|   IBIS model for TI AM261
[IBIS Ver]   5.1
[Disclaimer]   Please be aware that in the absence of a written agreement
|   Texas Instruments(TI) assumes no liability for:
|   (1) The accuracy of the IBIS models provided to your company,
|   however, the IBIS model is compliant to industry standard
|   IQ Level 2a.  Refer to IBIS Quality Section below for
|   for full details.
|   (2) The proper functioning of these Models in your design
|   or for any resulting applications
|   (3) Infringement of patents, copyrights or intellectual
|   property rights resulting from your use of these
|   models.
|   TI provides IBIS Models as a service to our customers and
|   therefore reserves the right to limit distribution of the
|   Models.  The information is subject to change without notice.
[File Name]  znc.ibs
[File Rev]   0.1
|   -Initial version
|   -Updated Package model
[Date]   10 October 2024
[Source]   Texas Instruments Incorporated
[Copyright]   Property of Texas Instruments Incorporated.
|   Unauthorized reproduction and/or distribution is strictly.
|   prohibited.
|   This product is protected under copyright law and trade
|   secret law as an unpublished work.
|   Created 2012,(C) Copyright 1999-2012,
|   Texas Instruments Incorporated., All Rights Reserved.
|   These commodities are under the U.S. Government
|   distribution license control. As such,they are not to be
|   re-exported without the prior approval of the U.S.
|   Department of Commerce.
[Notes]
   ADC pins are marked as NC
   USB pins are marked as NC
   Clock pins are marked as NC
   nReset pin marked as NC
|   Revision History
|   GERNERAL COMMENT: All IBIS Quality Notes below reflect latest release
|   and version of IBIS File
|   File passes ibischk6.0 with 0 errors and 35 warnings
|   Component AM261
[Component] AM261
[Manufacturer] TEXAS INSTRUMENTS
[Package Model] AM261_ZNC
[Package]
|   typ   min   max
R_pkg   0.1315   0.055671   0.23353
L_pkg   2.085e-9   9.776e-10   4.208e-9
C_pkg   2.503e-13   1.668e-13   9.865e-13
[Pin]   Signal_name   model_name
E6   VDD   POWER
E8   VDD   POWER
E10   VDD   POWER
E12   VDD   POWER
E14   VDD   POWER
F5   VDD   POWER
F15   VDD   POWER
H5   VDD   POWER
H15   VDD   POWER
K5   VDD   POWER
K15   VDD   POWER
M5   VDD   POWER
M15   VDD   POWER
P5   VDD   POWER
P15   VDD   POWER
R6   VDD   POWER
R15   VDD   POWER
T6   VDD   POWER
U9   VDDA18_LDO   POWER
U7   VDDA18_OSC_PLL   POWER
U3   VDDA18_USB   POWER
T10   VDDA33   POWER
T12   VDDA33   POWER
R3   VDDA33_USB   POWER
C11   VDDAR2   POWER
G3   VDDAR3   POWER
D6   VDDS18   POWER
D10   VDDS18   POWER
D14   VDDS18   POWER
H4   VDDS18   POWER
H16   VDDS18   POWER
L3   VDDS18   POWER
M16   VDDS18   POWER
T16   VDDS18   POWER
V4   VDDS18_LDO   POWER
C15   VDDSHV_A   POWER
D8   VDDSHV_A   POWER
D12   VDDSHV_A   POWER
F4   VDDSHV_A   POWER
F16   VDDSHV_A   POWER
K16   VDDSHV_A   POWER
P4   VDDSHV_B   POWER
T14   VDDSHV_C   POWER
K4   VDDSHV_D   POWER
M4   VDDSHV_D   POWER
P16   VDDSHV_E   POWER
U5   VDDSHV_F   POWER
T8   VDD_TEMP   NC
J17   VNWA   POWER
N3   VPP   POWER
W12   ADC0_AIN0   NC
V12   ADC0_AIN1   NC
V13   ADC0_AIN2   NC
U11   ADC0_AIN3   NC
W13   ADC0_AIN4   NC
U13   ADC0_AIN5   NC
W14   ADC0_AIN6   NC
W8   ADC2_AIN0   NC
V9   ADC2_AIN1   NC
V6   ADC2_AIN2   NC
V7   ADC2_AIN3   NC
W9   ADC2_AIN4   NC
V8   ADC2_AIN5   NC
W7   ADC2_AIN6   NC
U15   ADC_CAL0   NC
V11   ADC_VREFHI_G0   NC
V10   ADC_VREFHI_G1   NC
W11   ADC_VREFLO_G0   NC
W10   ADC_VREFLO_G1   NC
W5   ATESTV1   NC
W6   DAC_OUT   NC
V14   DAC_VREF0   NC
R1   GPIO0   bc1833dv40dcpbfbp18ll_rxll_ssdlv
R2   GPIO1   bc1833dv40dcpbfbp18ll_rxll_ssdlv
M2   GPIO2   bc1833dv40dcpbfbp18ll_rxll_ssdlv
N2   GPIO3   bc1833dv40dcpbfbp18ll_ssdlv
N1   GPIO4   bc1833dv40dcpbfbp18ll_ssdlv
P2   GPIO5   bc1833dv40dcpbfbp18ll_rxll_ssdlv
P1   GPIO6   bc1833dv40dcpbfbp18ll_rxll_ssdlv
K2   GPIO7   bc1833dv40dcpbfbp18ll_rxll_ssdlv
L1   GPIO8   bc1833dv40dcpbfbp18ll_rxll_ssdlv
J2   GPIO9   bc1833dv40dcpbfbp18ll_rxll_ssdlv
K1   GPIO10   bc1833dv40dcpbfbp18ll_rxll_ssdlv
C13   GPIO11   bc1833dv40dcpbfbp18ll_rxll_ssdlh
A12   GPIO12   bc1833dv40dcpbfbp18ll_ssdlh
B12   GPIO13   bc1833dv40dcpbfbp18ll_ssdlh
B11   GPIO14   bc1833dv40dcpbfbp18ll_rxll_ssdlh
A11   GPIO19   bc1833dv40dcpbfbp18ll_rxll_ssdlh
B10   GPIO20   bc1833dv40dcpbfbp18ll_rxll_ssdlh
A10   GPIO21   bc1833dv40dcpbfbp18ll_rxll_ssdlh
B9   GPIO22   bc1833dv40dcpbfbp18ll_rxll_ssdlh
C9   GPIO25   bc1833dv40dcpbfbp18ll_rxll_ssdlh
A9   GPIO26   bc1833dv40dcpbfbp18ll_rxll_ssdlh
A8   GPIO27   bc1833dv40dcpbfbp18ll_rxll_ssdlh
B8   GPIO28   bc1833dv40dcpbfbp18ll_rxll_ssdlh
V19   GPIO29   bc1833dv40dcpbfbp18ll_rxll_ssdlv_135u
U17   GPIO30   bc1833dv40dcpbfbp18ll_rxll_ssdlv_135u
W17   GPIO31   bc1833dv40dcpbfbp18ll_rxll_ssdlh
V17   GPIO32   bc1833dv40dcpbfbp18ll_rxll_ssdlh
W18   GPIO33   bc1833dv40dcpbfbp18ll_rxll_ssdlh
V18   GPIO34   bc1833dv40dcpbfbp18ll_rxll_ssdlv_135u
R18   GPIO35   bc1833dv40dcpbfbp18ll_rxll_ssdlv_135u
T19   GPIO36   bc1833dv40dcpbfbp18ll_rxll_ssdlv_135u
U18   GPIO37   bc1833dv40dcpbfbp18ll_rxll_ssdlv_135u
U19   GPIO38   bc1833dv40dcpbfbp18ll_rxll_ssdlv_135u
R17   GPIO39   bc1833dv40dcpbfbp18ll_rxll_ssdlv_135u
T18   GPIO40   bc1833dv40dcpbfbp18ll_rxll_ssdlv_135u
P18   GPIO41   bc1833dv40dcpbfbp18ll_rxll_ssdlv_135u
R19   GPIO42   bc1833dv40dcpbfbp18ll_rxll_ssdlv_135u
B5   GPIO43   bc1833dv40dcpbfbp18ll_rxll_ssdlh_135u
A6   GPIO44   bc1833dv40dcpbfbp18ll_rxll_ssdlh_135u
A5   GPIO45   bc1833dv40dcpbfbp18ll_rxll_ssdlh_135u
A4   GPIO46   bc1833dv40dcpbfbp18ll_rxll_ssdlh_135u
A3   GPIO47   bc1833dv40dcpbfbp18ll_rxll_ssdlh_135u
B4   GPIO48   bc1833dv40dcpbfbp18ll_rxll_ssdlh_135u
A2   GPIO49   bc1833dv40dcpbfbp18ll_rxll_ssdlh_135u
B2   GPIO50   bc1833dv40dcpbfbp18ll_rxll_ssdlv
B1   GPIO51   bc1833dv40dcpbfbp18ll_rxll_ssdlv
B3   GPIO52   bc1833dv40dcpbfbp18ll_rxll_ssdlv
C2   GPIO53   bc1833dv40dcpbfbp18ll_rxll_ssdlv
C1   GPIO54   bc1833dv40dcpbfbp18ll_rxll_ssdlv
E3   GPIO55   bc1833dv40dcpbfbp18ll_rxll_ssdlv
E2   GPIO56   bc1833dv40dcpbfbp18ll_rxll_ssdlv
D2   GPIO57   bc1833dv40dcpbfbp18ll_rxll_ssdlv
D1   GPIO58   bc1833dv40dcpbfbp18ll_rxll_ssdlv
E1   GPIO59   bc1833dv40dcpbfbp18ll_rxll_ssdlv
F1   GPIO60   bc1833dv40dcpbfbp18ll_rxll_ssdlv
F2   GPIO61   bc1833dv40dcpbfbp18ll_rxll_ssdlv
G1   GPIO62   bc1833dv40dcpbfbp18ll_rxll_ssdlv
G2   GPIO67   bc1833dv40dcpbfbp18ll_rxll_ssdlv
H1   GPIO68   bc1833dv40dcpbfbp18ll_rxll_ssdlv
H2   GPIO69   bc1833dv40dcpbfbp18ll_rxll_ssdlv
J1   GPIO70   bc1833dv40dcpbfbp18ll_rxll_ssdlv
V15   GPIO71   bc1833dv40dcpbfbp18ll_rxll_ssdlh
W15   GPIO72   bc1833dv40dcpbfbp18ll_rxll_ssdlh
W16   GPIO73   bc1833dv40dcpbfbp18ll_rxll_ssdlh
V16   GPIO74   bc1833dv40dcpbfbp18ll_rxll_ssdlh
L2   GPIO75   bc1833dv40dcpbfbp18ll_rxll_ssdlv
M1   GPIO76   bc1833dv40dcpbfbp18ll_rxll_ssdlv
N17   GPIO85   bc1833dv40dcpbfbp18ll_rxll_ssdlv_135u
P19   GPIO86   bc1833dv40dcpbfbp18ll_rxll_ssdlv_135u
G17   GPIO87   bc1833dv40dcpbfbp18ll_rxll_ssdlv_135u
J18   GPIO89   bc1833dv40dcpbfbp18ll_rxll_ssdlv_135u
G19   GPIO90   bc1833dv40dcpbfbp18ll_rxll_ssdlv_135u
L18   GPIO91   bc1833dv40dcpbfbp18ll_rxll_ssdlv_135u
J19   GPIO92   bc1833dv40dcpbfbp18ll_rxll_ssdlv_135u
M18   GPIO93   bc1833dv40dcpbfbp18ll_rxll_ssdlv_135u
L19   GPIO94   bc1833dv40dcpbfbp18ll_rxll_ssdlv_135u
K19   GPIO95   bc1833dv40dcpbfbp18ll_rxll_ssdlv_135u
L17   GPIO96   bc1833dv40dcpbfbp18ll_rxll_ssdlv_135u
K18   GPIO97   bc1833dv40dcpbfbp18ll_rxll_ssdlv_135u
M19   GPIO98   bc1833dv40dcpbfbp18ll_rxll_ssdlv_135u
N18   GPIO99   bc1833dv40dcpbfbp18ll_rxll_ssdlv_135u
N19   GPIO100   bc1833dv40dcpbfbp18ll_rxll_ssdlv_135u
H19   GPIO101   bc1833dv40dcpbfbp18ll_rxll_ssdlv_135u
H18   GPIO102   bc1833dv40dcpbfbp18ll_rxll_ssdlv_135u
E18   GPIO103   bc1833dv40dcpbfbp18ll_rxll_ssdlv_135u
C19   GPIO106   bc1833dv40dcpbfbp18ll_rxll_ssdlv_135u
D19   GPIO107   bc1833dv40dcpbfbp18ll_rxll_ssdlv_135u
E19   GPIO108   bc1833dv40dcpbfbp18ll_rxll_ssdlv_135u
G18   GPIO109   bc1833dv40dcpbfbp18ll_rxll_ssdlv_135u
F18   GPIO110   bc1833dv40dcpbfbp18ll_rxll_ssdlv_135u
E17   GPIO111   bc1833dv40dcpbfbp18ll_rxll_ssdlv_135u
F19   GPIO112   bc1833dv40dcpbfbp18ll_rxll_ssdlv_135u
B18   GPIO113   bc1833dv40dcpbfbp18ll_rxll_ssdlv_135u
A18   GPIO114   bc1833dv40dcpbfbp18ll_rxll_ssdlv_135u
D18   GPIO115   bc1833dv40dcpbfbp18ll_rxll_ssdlv_135u
C18   GPIO116   bc1833dv40dcpbfbp18ll_rxll_ssdlv_135u
B19   GPIO117   bc1833dv40dcpbfbp18ll_rxll_ssdlv_135u
C17   GPIO118   bc1833dv40dcpbfbp18ll_rxll_ssdlv_135u
B16   GPIO119   bc1833dv40dcpbfbp18ll_rxll_ssdlh
B17   GPIO120   bc1833dv40dcpbfbp18ll_rxll_ssdlv_135u
T1   GPIO121   bc1833dv40dcpbfbp18ll_rxll_ssdlh
A17   GPIO126   bc1833dv40dcpbfbp18ll_rxll_ssdlh
A16   GPIO127   bc1833dv40dcpbfbp18ll_rxll_ssdlh
B15   GPIO130   bc1833dv40dcpbfbp18ll_rxll_ssdlh
A15   GPIO131   bc1833dv40dcpbfbp18ll_rxll_ssdlh
A14   GPIO132   bc1833dv40dcpbfbp18ll_rxll_ssdlh
B14   GPIO133   bc1833dv40dcpbfbp18ll_rxll_ssdlh
B13   GPIO134   bi2c1833dvfzp18_ssdlh
A13   GPIO135   bi2c1833dvfzp18_ssdlh
J3   GPIO138   bc1833dv40dcpbfbp18ll_rxll_ssdlv
V1   GPIO139   NC
U1   GPIO140   NC
T2   PORZ   ihhv1833dvhyp18ll_ssdhv
C5   SAFETY_ERRORN   bc1833dv40dcpbfbp18ll_ssdlh_135u
B6   TCK   iq1833dvtckpbfbp18ll_ssdhh_135u
C7   TDI   bc1833dv40dcpbfbp18ll_ssdlh_135u
A7   TDO   bc1833dv40dcpbfbp18ll_ssdlh_135u
W4   TEMPCAL   NC
B7   TMS   bc1833dv40dcpbfbp18ll_ssdlh_135u
V5   VSYS_MON   NC
C3   WARMRSTN   bc1833dv40dcpbfbp18ll_od_fs_cmphdl_ssdlv
W3   XTAL_XI   NC
W2   XTAL_XO   NC
A1   VSS   GND
A19   VSS   GND
D4   VSS   GND
D16   VSS   GND
E5   VSS   GND
E15   VSS   GND
F6   VSS   GND
F7   VSS   GND
F8   VSS   GND
F9   VSS   GND
F10   VSS   GND
F11   VSS   GND
F12   VSS   GND
F13   VSS   GND
F14   VSS   GND
G6   VSS   GND
G7   VSS   GND
G8   VSS   GND
G9   VSS   GND
G10   VSS   GND
G11   VSS   GND
G12   VSS   GND
G13   VSS   GND
G14   VSS   GND
H6   VSS   GND
H7   VSS   GND
H8   VSS   GND
H9   VSS   GND
H10   VSS   GND
H11   VSS   GND
H12   VSS   GND
H13   VSS   GND
H14   VSS   GND
J6   VSS   GND
J7   VSS   GND
J8   VSS   GND
J9   VSS   GND
J10   VSS   GND
J11   VSS   GND
J12   VSS   GND
J13   VSS   GND
J14   VSS   GND
K6   VSS   GND
K7   VSS   GND
K8   VSS   GND
K9   VSS   GND
K10   VSS   GND
K11   VSS   GND
K12   VSS   GND
K13   VSS   GND
K14   VSS   GND
L6   VSS   GND
L7   VSS   GND
L8   VSS   GND
L9   VSS   GND
L10   VSS   GND
L11   VSS   GND
L12   VSS   GND
L13   VSS   GND
L14   VSS   GND
M6   VSS   GND
M7   VSS   GND
M8   VSS   GND
M9   VSS   GND
M10   VSS   GND
M11   VSS   GND
M12   VSS   GND
M13   VSS   GND
M14   VSS   GND
N6   VSS   GND
N7   VSS   GND
N8   VSS   GND
N9   VSS   GND
N10   VSS   GND
N11   VSS   GND
N12   VSS   GND
N13   VSS   GND
N14   VSS   GND
P6   VSS   GND
P7   VSS   GND
P8   VSS   GND
P9   VSS   GND
P10   VSS   GND
P11   VSS   GND
P12   VSS   GND
P13   VSS   GND
P14   VSS   GND
R5   VSS   GND
R8   VSS   GND
R14   VSS   GND
T4   VSS   GND
U2   VSS   GND
V2   VSS   GND
V3   VSS   GND
W1   VSS   GND
W19   VSS   GND
R10   VSSA   GND
R12   VSSA   GND
|   BC1833DV40DCPBFBP18LL_SSDLH
[Model Selector] bc1833dv40dcpbfbp18ll_ssdlh
|SC1 IS A SLEW RATE CONTROL PIN
|5% SUPPLY VARIATION MODES WITH 1.8V NOM SUPPLY
BC40D_H_PUPDOFF_5P_SC1_1P8  Cell operated at 1.8(nom)
|BC40D_H_PUPDOFF_5P_SC1_1P8; BUFFER WITH WEAK PULUP/PULLDOWN OFF AT 5% SUPPLY
|VARIATION WITH SC1=1 MEANING SLOW MODE OF OPERATION
BC40D_H_PD_ON_5P_!SC1_1P8  Cell operated at 1.8(nom)
|BC40D_H_PD_ON_5P_!SC1_1P8; BUFFER WITH WEAK_PULLDOWN_ON AT 5% SUPPLY
|VARIATION WITH SC1=0 MEANING FAST MODE OF OPERATION
BC40D_H_PD_ON_5P_SC1_1P8  Cell operated at 1.8(nom)
|BC40D_H_PD_ON_5P_SC1_1P8; BUFFER WITH WEAK_PULLDOWN_ON AT 5% SUPPLY
|VARIATION WITH SC1=1 MEANING SLOW MODE OF OPERATION
BC40D_H_PU_ON_5P_!SC1_1P8  Cell operated at 1.8(nom)
|BC40D_H_PU_ON_5P_!SC1_1P8; BUFFER WITH WEAK_PULLUP_ON AT 5% SUPPLY
|VARIATION WITH SC1=0 MEANING FAST MODE OF OPERATION
BC40D_H_PUPDOFF_5P_!SC1_1P8  Cell operated at 1.8(nom)
|BC40D_H_PUPDOFF_5P_!SC1_1P8; BUFFER WITH WEAK PULUP/PULLDOWN OFF AT 5% SUPPLY
|VARIATION WITH SC1=0 MEANING FAST MODE OF OPERATION
BC40D_H_PU_ON_5P_SC1_1P8  Cell operated at 1.8(nom)
|BC40D_H_PU_ON_5P_SC1_1P8; BUFFER WITH WEAK_PULLUP_ON AT 5% SUPPLY
|VARIATION WITH SC1=1 MEANING SLOW MODE OF OPERATION
|5% SUPPLY VARIATION MODES WITH 3.3V NOM SUPPLY
BC40D_H_PUPDOFF_5P_SC1_3P3  Cell operated at 3.3(nom)
|BC40D_H_PUPDOFF_5P_SC1_3P3; BUFFER WITH WEAK PULUP/PULLDOWN OFF AT 5% SUPPLY
|VARIATION WITH SC1=1 MEANING SLOW MODE OF OPERATION
BC40D_H_PD_ON_5P_!SC1_3P3  Cell operated at 3.3(nom)
|BC40D_H_PD_ON_5P_!SC1_3P3; BUFFER WITH WEAK_PULLDOWN_ON AT 5% SUPPLY
|VARIATION WITH SC1=0 MEANING FAST MODE OF OPERATION
BC40D_H_PD_ON_5P_SC1_3P3  Cell operated at 3.3(nom)
|BC40D_H_PD_ON_5P_SC1_3P3; BUFFER WITH WEAK_PULLDOWN_ON AT 5% SUPPLY
|VARIATION WITH SC1=1 MEANING SLOW MODE OF OPERATION
BC40D_H_PU_ON_5P_!SC1_3P3  Cell operated at 3.3(nom)
|BC40D_H_PU_ON_5P_!SC1_3P3; BUFFER WITH WEAK_PULLUP_ON AT 5% SUPPLY
|VARIATION WITH SC1=0 MEANING FAST MODE OF OPERATION
BC40D_H_PUPDOFF_5P_!SC1_3P3  Cell operated at 3.3(nom)
|BC40D_H_PUPDOFF_5P_!SC1_3P3; BUFFER WITH WEAK PULUP/PULLDOWN OFF AT 5% SUPPLY
|VARIATION WITH SC1=0 MEANING FAST MODE OF OPERATION
BC40D_H_PU_ON_5P_SC1_3P3  Cell operated at 3.3(nom)
|BC40D_H_PU_ON_5P_SC1_3P3; BUFFER WITH WEAK_PULLUP_ON AT 5% SUPPLY
|VARIATION WITH SC1=1 MEANING SLOW MODE OF OPERATION
| 10% SUPPLY VARIATION MODES WITH 1.8V NOM SUPPLY
BC40D_H_PUPDOFF_10P_SC1_1P8  Cell operated at 1.8(nom)
|BC40D_H_PUPDOFF_10P_SC1_1P8; BUFFER WITH WEAK PULUP/PULLDOWN OFF AT 10% SUPPLY
|VARIATION WITH SC1=1 MEANING SLOW MODE OF OPERATION
BC40D_H_PD_ON_10P_!SC1_1P8  Cell operated at 1.8(nom)
|BC40D_H_PD_ON_10P_!SC1_1P8; BUFFER WITH WEAK_PULLDOWN_ON AT 10% SUPPLY
|VARIATION WITH SC1=0 MEANING FAST MODE OF OPERATION
BC40D_H_PD_ON_10P_SC1_1P8  Cell operated at 1.8(nom)
|BC40D_H_PD_ON_10P_SC1_1P8; BUFFER WITH WEAK_PULLDOWN_ON AT 10% SUPPLY
|VARIATION WITH SC1=1 MEANING SLOW MODE OF OPERATION
BC40D_H_PU_ON_10P_!SC1_1P8  Cell operated at 1.8(nom)
|BC40D_H_PU_ON_10P_!SC1_1P8; BUFFER WITH WEAK_PULLUP_ON AT 10% SUPPLY
|VARIATION WITH SC1=0 MEANING FAST MODE OF OPERATION
BC40D_H_PUPDOFF_10P_!SC1_1P8  Cell operated at 1.8(nom)
|BC40D_H_PUPDOFF_10P_!SC1_1P8; BUFFER WITH WEAK PULUP/PULLDOWN OFF AT 10% SUPPLY
|VARIATION WITH SC1=0 MEANING FAST MODE OF OPERATION
BC40D_H_PU_ON_10P_SC1_1P8  Cell operated at 1.8(nom)
|BC40D_H_PU_ON_10P_SC1_1P8; BUFFER WITH WEAK_PULLUP_ON AT 10% SUPPLY
|VARIATION WITH SC1=1 MEANING SLOW MODE OF OPERATION
| 10% SUPPLY VARIATION MODES WITH 3.3V NOM SUPPLY
BC40D_H_PUPDOFF_10P_SC1_3P3  Cell operated at 3.3(nom)
|BC40D_H_PUPDOFF_10P_SC1_3P3; BUFFER WITH WEAK PULUP/PULLDOWN OFF AT 10% SUPPLY
|VARIATION WITH SC1=1 MEANING SLOW MODE OF OPERATION
BC40D_H_PD_ON_10P_!SC1_3P3  Cell operated at 3.3(nom)
|BC40D_H_PD_ON_10P_!SC1_3P3; BUFFER WITH WEAK_PULLDOWN_ON 10% SUPPLY
|VARIATION WITH SC1=0 MEANING FAST MODE OF OPERATION
BC40D_H_PD_ON_10P_SC1_3P3  Cell operated at 3.3(nom)
|BC40D_H_PD_ON_10P_SC1_3P3; BUFFER WITH WEAK_PULLDOWN_ON AT 10% SUPPLY
|VARIATION WITH SC1=1 MEANING SLOW MODE OF OPERATION
BC40D_H_PU_ON_10P_!SC1_3P3  Cell operated at 3.3(nom)
|BC40D_H_PU_ON_10P_!SC1_3P3; BUFFER WITH WEAK_PULLUP_ON AT 10% SUPPLY
|VARIATION WITH SC1=0 MEANING FAST MODE OF OPERATION
BC40D_H_PUPDOFF_10P_!SC1_3P3  Cell operated at 3.3(nom)
|BC40D_H_PUPDOFF_10P_!SC1_3P3; BUFFER WITH WEAK PULUP/PULLDOWN OFF AT 10% SUPPLY
|VARIATION WITH SC1=0 MEANING FAST MODE OF OPERATION
BC40D_H_PU_ON_10P_SC1_3P3  Cell operated at 3.3(nom)
|BC40D_H_PU_ON_10P_SC1_3P3; BUFFER WITH WEAK_PULLUP_ON AT 10% SUPPLY
|VARIATION WITH SC1=1 MEANING SLOW MODE OF OPERATION
|   BC1833DV40DCPBFBP18LL_SSDLV
[Model Selector] bc1833dv40dcpbfbp18ll_ssdlv
|SC1 IS A SLEW RATE CONTROL PIN
|5% SUPPLY VARIATION MODES WITH 1.8V NOM SUPPLY
BC40D_V_PUPDOFF_5P_SC1_1P8  Cell operated at 1.8(nom)
|BC40D_V_PUPDOFF_5P_SC1_1P8; BUFFER WITH WEAK PULUP/PULLDOWN OFF AT 5% SUPPLY
|VARIATION WITH SC1=1 MEANING SLOW MODE OF OPERATION
BC40D_V_PD_ON_5P_!SC1_1P8  Cell operated at 1.8(nom)
|BC40D_V_PD_ON_5P_!SC1_1P8; BUFFER WITH WEAK_PULLDOWN_ON AT 5% SUPPLY
|VARIATION WITH SC1=0 MEANING FAST MODE OF OPERATION
BC40D_V_PD_ON_5P_SC1_1P8  Cell operated at 1.8(nom)
|BC40D_V_PD_ON_5P_SC1_1P8; BUFFER WITH WEAK_PULLDOWN_ON AT 5% SUPPLY
|VARIATION WITH SC1=1 MEANING SLOW MODE OF OPERATION
BC40D_V_PU_ON_5P_!SC1_1P8  Cell operated at 1.8(nom)
|BC40D_V_PU_ON_5P_!SC1_1P8; BUFFER WITH WEAK_PULLUP_ON AT 5% SUPPLY
|VARIATION WITH SC1=0 MEANING FAST MODE OF OPERATION
BC40D_V_PUPDOFF_5P_!SC1_1P8  Cell operated at 1.8(nom)
|BC40D_V_PUPDOFF_5P_!SC1_1P8; BUFFER WITH WEAK PULUP/PULLDOWN OFF AT 5% SUPPLY
|VARIATION WITH SC1=0 MEANING FAST MODE OF OPERATION
BC40D_V_PU_ON_5P_SC1_1P8  Cell operated at 1.8(nom)
|BC40D_V_PU_ON_5P_SC1_1P8; BUFFER WITH WEAK_PULLUP_ON AT 5% SUPPLY
|VARIATION WITH SC1=1 MEANING SLOW MODE OF OPERATION
|5% SUPPLY VARIATION MODES WITH 3.3V NOM SUPPLY
BC40D_V_PUPDOFF_5P_SC1_3P3  Cell operated at 3.3(nom)
|BC40D_V_PUPDOFF_5P_SC1_3P3; BUFFER WITH WEAK PULUP/PULLDOWN OFF AT 5% SUPPLY
|VARIATION WITH SC1=1 MEANING SLOW MODE OF OPERATION
BC40D_V_PD_ON_5P_!SC1_3P3  Cell operated at 3.3(nom)
|BC40D_V_PD_ON_5P_!SC1_3P3; BUFFER WITH WEAK_PULLDOWN_ON AT 5% SUPPLY
|VARIATION WITH SC1=0 MEANING FAST MODE OF OPERATION
BC40D_V_PD_ON_5P_SC1_3P3  Cell operated at 3.3(nom)
|BC40D_V_PD_ON_5P_SC1_3P3; BUFFER WITH WEAK_PULLDOWN_ON AT 5% SUPPLY
|VARIATION WITH SC1=1 MEANING SLOW MODE OF OPERATION
BC40D_V_PU_ON_5P_!SC1_3P3  Cell operated at 3.3(nom)
|BC40D_V_PU_ON_5P_!SC1_3P3; BUFFER WITH WEAK_PULLUP_ON AT 5% SUPPLY
|VARIATION WITH SC1=0 MEANING FAST MODE OF OPERATION
BC40D_V_PUPDOFF_5P_!SC1_3P3  Cell operated at 3.3(nom)
|BC40D_V_PUPDOFF_5P_!SC1_3P3; BUFFER WITH WEAK PULUP/PULLDOWN OFF AT 5% SUPPLY
|VARIATION WITH SC1=0 MEANING FAST MODE OF OPERATION
BC40D_V_PU_ON_5P_SC1_3P3  Cell operated at 3.3(nom)
|BC40D_V_PU_ON_5P_SC1_3P3; BUFFER WITH WEAK_PULLUP_ON AT 5% SUPPLY
|VARIATION WITH SC1=1 MEANING SLOW MODE OF OPERATION
| 10% SUPPLY VARIATION MODES WITH 1.8V NOM SUPPLY
BC40D_V_PUPDOFF_10P_SC1_1P8  Cell operated at 1.8(nom)
|BC40D_V_PUPDOFF_10P_SC1_1P8; BUFFER WITH WEAK PULUP/PULLDOWN OFF AT 10% SUPPLY
|VARIATION WITH SC1=1 MEANING SLOW MODE OF OPERATION
BC40D_V_PD_ON_10P_!SC1_1P8  Cell operated at 1.8(nom)
|BC40D_V_PD_ON_10P_!SC1_1P8; BUFFER WITH WEAK_PULLDOWN_ON AT 10% SUPPLY
|VARIATION WITH SC1=0 MEANING FAST MODE OF OPERATION
BC40D_V_PD_ON_10P_SC1_1P8  Cell operated at 1.8(nom)
|BC40D_V_PD_ON_10P_SC1_1P8; BUFFER WITH WEAK_PULLDOWN_ON AT 10% SUPPLY
|VARIATION WITH SC1=1 MEANING SLOW MODE OF OPERATION
BC40D_V_PU_ON_10P_!SC1_1P8  Cell operated at 1.8(nom)
|BC40D_V_PU_ON_10P_!SC1_1P8; BUFFER WITH WEAK_PULLUP_ON AT 10% SUPPLY
|VARIATION WITH SC1=0 MEANING FAST MODE OF OPERATION
BC40D_V_PUPDOFF_10P_!SC1_1P8  Cell operated at 1.8(nom)
|BC40D_V_PUPDOFF_10P_!SC1_1P8; BUFFER WITH WEAK PULUP/PULLDOWN OFF AT 10% SUPPLY
|VARIATION WITH SC1=0 MEANING FAST MODE OF OPERATION
BC40D_V_PU_ON_10P_SC1_1P8  Cell operated at 1.8(nom)
|BC40D_V_PU_ON_10P_SC1_1P8; BUFFER WITH WEAK_PULLUP_ON AT 10% SUPPLY
|VARIATION WITH SC1=1 MEANING SLOW MODE OF OPERATION
| 10% SUPPLY VARIATION MODES WITH 3.3V NOM SUPPLY
BC40D_V_PUPDOFF_10P_SC1_3P3  Cell operated at 3.3(nom)
|BC40D_V_PUPDOFF_10P_SC1_3P3; BUFFER WITH WEAK PULUP/PULLDOWN OFF AT 10% SUPPLY
|VARIATION WITH SC1=1 MEANING SLOW MODE OF OPERATION
BC40D_V_PD_ON_10P_!SC1_3P3  Cell operated at 3.3(nom)
|BC40D_V_PD_ON_10P_!SC1_3P3; BUFFER WITH WEAK_PULLDOWN_ON 10% SUPPLY
|VARIATION WITH SC1=0 MEANING FAST MODE OF OPERATION
BC40D_V_PD_ON_10P_SC1_3P3  Cell operated at 3.3(nom)
|BC40D_V_PD_ON_10P_SC1_3P3; BUFFER WITH WEAK_PULLDOWN_ON AT 10% SUPPLY
|VARIATION WITH SC1=1 MEANING SLOW MODE OF OPERATION
BC40D_V_PU_ON_10P_!SC1_3P3  Cell operated at 3.3(nom)
|BC40D_V_PU_ON_10P_!SC1_3P3; BUFFER WITH WEAK_PULLUP_ON AT 10% SUPPLY
|VARIATION WITH SC1=0 MEANING FAST MODE OF OPERATION
BC40D_V_PUPDOFF_10P_!SC1_3P3  Cell operated at 3.3(nom)
|BC40D_V_PUPDOFF_10P_!SC1_3P3; BUFFER WITH WEAK PULUP/PULLDOWN OFF AT 10% SUPPLY
|VARIATION WITH SC1=0 MEANING FAST MODE OF OPERATION
BC40D_V_PU_ON_10P_SC1_3P3  Cell operated at 3.3(nom)
|BC40D_V_PU_ON_10P_SC1_3P3; BUFFER WITH WEAK_PULLUP_ON AT 10% SUPPLY
|VARIATION WITH SC1=1 MEANING SLOW MODE OF OPERATION
|   BI2C1833DVFZP18_SSDLH
[Model Selector] bi2c1833dvfzp18_ssdlh
BI2C1833_NORAML_5P_1P8  Cell operated at 1.8(nom)
|BI2C1833_NORAML_5P_1P8; I2C MODE AT 1.8V WITH 5% SUPPLY VARIATION
BI2C1833_NORAML_5P_3P3  Cell operated at 3.3(nom)
|BI2C1833_NORAML_5P_3P3; I2C MODE AT 3.3V WITH 5% SUPPLY VARIATION
BI2C1833_NORAML_10P_1P8  Cell operated at 1.8(nom)
|BI2C1833_NORAML_10P_1P8; I2C MODE AT 1.8V WITH 10% SUPPLY VARIATION
BI2C1833_NORAML_10P_3P3  Cell operated at 3.3(nom)
|BI2C1833_NORAML_10P_3P3; I2C MODE AT 3.3V WITH 10% SUPPLY VARIATION
|   IHHV1833DVHYP18LL_SSDHV
[Model Selector] ihhv1833dvhyp18ll_ssdhv
IHHV_NORAML_5P_1P8  Cell operated at 1.8(nom)
|IHHV_NORAML_5P_1P8; NORMAL MODE AT 1.8V WITH 5% SUPPLY VARIATION
IHHV_NORAML_5P_3P3  Cell operated at 3.3(nom)
|IHHV_NORAML_5P_3P3; NORMAL MODE AT 3.3V WITH 5% SUPPLY VARIATION
IHHV_NORAML_10P_1P8  Cell operated at 1.8(nom)
|IHHV_NORAML_10P_1P8; NORMAL MODE AT 1.8V WITH 10% SUPPLY VARIATION
IHHV_NORAML_10P_3P3  Cell operated at 3.3(nom)
|IHHV_NORAML_10P_3P3; NORMAL MODE AT 3.3V WITH 10% SUPPLY VARIATION
|   BC1833DV40DCPBFBP18LL_OD_FS_CMPHDL_SSDLV
[Model Selector] bc1833dv40dcpbfbp18ll_od_fs_cmphdl_ssdlv
|SC1 IS A SLEW RATE CONTROL PIN
|5% SUPPLY VARIATION MODES WITH 1.8V NOM SUPPLY
BC40D_V_PUPDOFF_5P_SC1_1P8  Cell operated at 1.8(nom)
|BC40D_V_PUPDOFF_5P_SC1_1P8; BUFFER WITH WEAK PULUP/PULLDOWN OFF AT 5% SUPPLY
|VARIATION WITH SC1=1 MEANING SLOW MODE OF OPERATION
BC40D_V_PD_ON_5P_!SC1_1P8  Cell operated at 1.8(nom)
|BC40D_V_PD_ON_5P_!SC1_1P8; BUFFER WITH WEAK_PULLDOWN_ON AT 5% SUPPLY
|VARIATION WITH SC1=0 MEANING FAST MODE OF OPERATION
BC40D_V_PD_ON_5P_SC1_1P8  Cell operated at 1.8(nom)
|BC40D_V_PD_ON_5P_SC1_1P8; BUFFER WITH WEAK_PULLDOWN_ON AT 5% SUPPLY
|VARIATION WITH SC1=1 MEANING SLOW MODE OF OPERATION
BC40D_V_PU_ON_5P_!SC1_1P8  Cell operated at 1.8(nom)
|BC40D_V_PU_ON_5P_!SC1_1P8; BUFFER WITH WEAK_PULLUP_ON AT 5% SUPPLY
|VARIATION WITH SC1=0 MEANING FAST MODE OF OPERATION
BC40D_V_PUPDOFF_5P_!SC1_1P8  Cell operated at 1.8(nom)
|BC40D_V_PUPDOFF_5P_!SC1_1P8; BUFFER WITH WEAK PULUP/PULLDOWN OFF AT 5% SUPPLY
|VARIATION WITH SC1=0 MEANING FAST MODE OF OPERATION
BC40D_V_PU_ON_5P_SC1_1P8  Cell operated at 1.8(nom)
|BC40D_V_PU_ON_5P_SC1_1P8; BUFFER WITH WEAK_PULLUP_ON AT 5% SUPPLY
|VARIATION WITH SC1=1 MEANING SLOW MODE OF OPERATION
|5% SUPPLY VARIATION MODES WITH 3.3V NOM SUPPLY
BC40D_V_PUPDOFF_5P_SC1_3P3  Cell operated at 3.3(nom)
|BC40D_V_PUPDOFF_5P_SC1_3P3; BUFFER WITH WEAK PULUP/PULLDOWN OFF AT 5% SUPPLY
|VARIATION WITH SC1=1 MEANING SLOW MODE OF OPERATION
BC40D_V_PD_ON_5P_!SC1_3P3  Cell operated at 3.3(nom)
|BC40D_V_PD_ON_5P_!SC1_3P3; BUFFER WITH WEAK_PULLDOWN_ON AT 5% SUPPLY
|VARIATION WITH SC1=0 MEANING FAST MODE OF OPERATION
BC40D_V_PD_ON_5P_SC1_3P3  Cell operated at 3.3(nom)
|BC40D_V_PD_ON_5P_SC1_3P3; BUFFER WITH WEAK_PULLDOWN_ON AT 5% SUPPLY
|VARIATION WITH SC1=1 MEANING SLOW MODE OF OPERATION
BC40D_V_PU_ON_5P_!SC1_3P3  Cell operated at 3.3(nom)
|BC40D_V_PU_ON_5P_!SC1_3P3; BUFFER WITH WEAK_PULLUP_ON AT 5% SUPPLY
|VARIATION WITH SC1=0 MEANING FAST MODE OF OPERATION
BC40D_V_PUPDOFF_5P_!SC1_3P3  Cell operated at 3.3(nom)
|BC40D_V_PUPDOFF_5P_!SC1_3P3; BUFFER WITH WEAK PULUP/PULLDOWN OFF AT 5% SUPPLY
|VARIATION WITH SC1=0 MEANING FAST MODE OF OPERATION
BC40D_V_PU_ON_5P_SC1_3P3  Cell operated at 3.3(nom)
|BC40D_V_PU_ON_5P_SC1_3P3; BUFFER WITH WEAK_PULLUP_ON AT 5% SUPPLY
|VARIATION WITH SC1=1 MEANING SLOW MODE OF OPERATION
| 10% SUPPLY VARIATION MODES WITH 1.8V NOM SUPPLY
BC40D_V_PUPDOFF_10P_SC1_1P8  Cell operated at 1.8(nom)
|BC40D_V_PUPDOFF_10P_SC1_1P8; BUFFER WITH WEAK PULUP/PULLDOWN OFF AT 10% SUPPLY
|VARIATION WITH SC1=1 MEANING SLOW MODE OF OPERATION
BC40D_V_PD_ON_10P_!SC1_1P8  Cell operated at 1.8(nom)
|BC40D_V_PD_ON_10P_!SC1_1P8; BUFFER WITH WEAK_PULLDOWN_ON AT 10% SUPPLY
|VARIATION WITH SC1=0 MEANING FAST MODE OF OPERATION
BC40D_V_PD_ON_10P_SC1_1P8  Cell operated at 1.8(nom)
|BC40D_V_PD_ON_10P_SC1_1P8; BUFFER WITH WEAK_PULLDOWN_ON AT 10% SUPPLY
|VARIATION WITH SC1=1 MEANING SLOW MODE OF OPERATION
BC40D_V_PU_ON_10P_!SC1_1P8  Cell operated at 1.8(nom)
|BC40D_V_PU_ON_10P_!SC1_1P8; BUFFER WITH WEAK_PULLUP_ON AT 10% SUPPLY
|VARIATION WITH SC1=0 MEANING FAST MODE OF OPERATION
BC40D_V_PUPDOFF_10P_!SC1_1P8  Cell operated at 1.8(nom)
|BC40D_V_PUPDOFF_10P_!SC1_1P8; BUFFER WITH WEAK PULUP/PULLDOWN OFF AT 10% SUPPLY
|VARIATION WITH SC1=0 MEANING FAST MODE OF OPERATION
BC40D_V_PU_ON_10P_SC1_1P8  Cell operated at 1.8(nom)
|BC40D_V_PU_ON_10P_SC1_1P8; BUFFER WITH WEAK_PULLUP_ON AT 10% SUPPLY
|VARIATION WITH SC1=1 MEANING SLOW MODE OF OPERATION
| 10% SUPPLY VARIATION MODES WITH 3.3V NOM SUPPLY
BC40D_V_PUPDOFF_10P_SC1_3P3  Cell operated at 3.3(nom)
|BC40D_V_PUPDOFF_10P_SC1_3P3; BUFFER WITH WEAK PULUP/PULLDOWN OFF AT 10% SUPPLY
|VARIATION WITH SC1=1 MEANING SLOW MODE OF OPERATION
BC40D_V_PD_ON_10P_!SC1_3P3  Cell operated at 3.3(nom)
|BC40D_V_PD_ON_10P_!SC1_3P3; BUFFER WITH WEAK_PULLDOWN_ON 10% SUPPLY
|VARIATION WITH SC1=0 MEANING FAST MODE OF OPERATION
BC40D_V_PD_ON_10P_SC1_3P3  Cell operated at 3.3(nom)
|BC40D_V_PD_ON_10P_SC1_3P3; BUFFER WITH WEAK_PULLDOWN_ON AT 10% SUPPLY
|VARIATION WITH SC1=1 MEANING SLOW MODE OF OPERATION
BC40D_V_PU_ON_10P_!SC1_3P3  Cell operated at 3.3(nom)
|BC40D_V_PU_ON_10P_!SC1_3P3; BUFFER WITH WEAK_PULLUP_ON AT 10% SUPPLY
|VARIATION WITH SC1=0 MEANING FAST MODE OF OPERATION
BC40D_V_PUPDOFF_10P_!SC1_3P3  Cell operated at 3.3(nom)
|BC40D_V_PUPDOFF_10P_!SC1_3P3; BUFFER WITH WEAK PULUP/PULLDOWN OFF AT 10% SUPPLY
|VARIATION WITH SC1=0 MEANING FAST MODE OF OPERATION
BC40D_V_PU_ON_10P_SC1_3P3  Cell operated at 3.3(nom)
|BC40D_V_PU_ON_10P_SC1_3P3; BUFFER WITH WEAK_PULLUP_ON AT 10% SUPPLY
|VARIATION WITH SC1=1 MEANING SLOW MODE OF OPERATION
|   IQ1833DVTCKPBFBP18LL_SSDHH_135U
[Model Selector] iq1833dvtckpbfbp18ll_ssdhh_135u
|5% SUPPLY VARIATION MODES WITH 1.8V NOM SUPPLY
IQ_SSDHH_PD_ON_5P_1P8  Cell operated at 1.8(nom)
|IQ_SSDHH_PD_ON_5P_1P8; BUFFER WITH WEAK_PULLDOWN_ON AT 5% SUPPLY VARIATION
IQ_SSDHH_PU_ON_5P_1P8  Cell operated at 1.8(nom)
|IQ_SSDHH_PU_ON_5P_1P8; BUFFER WITH WEAK_PULLUP_ON AT 5% SUPPLY VARIATION
IQ_SSDHH_PUPDOFF_5P_1P8  Cell operated at 1.8(nom)
|IQ_SSDHH_PUPDOFF_5P_1P8; BUFFER WITH WEAK PUPD OFF AT 5% SUPPLY VARIATION
|5% SUPPLY VARIATION MODES WITH 3.3V NOM SUPPLY
IQ_SSDHH_PD_ON_5P_3P3  Cell operated at 3.3(nom)
|IQ_SSDHH_PD_ON_5P_3P3; BUFFER WITH WEAK_PULLDOWN_ON AT 5% SUPPLY VARIATION
IQ_SSDHH_PU_ON_5P_3P3  Cell operated at 3.3(nom)
|IQ_SSDHH_PU_ON_5P_3P3; BUFFER WITH WEAK_PULLUP_ON AT 5% SUPPLY VARIATION
IQ_SSDHH_PUPDOFF_5P_3P3  Cell operated at 3.3(nom)
|IQ_SSDHH_PUPDOFF_5P_3P3; BUFFER WITH WEAK PUPD OFF AT 5% SUPPLY VARIATION
|10% SUPPLY VARIATION MODES WITH 1.8V NOM SUPPLY
IQ_SSDHH_PD_ON_10P_1P8  Cell operated at 1.8(nom)
|IQ_SSDHH_PD_ON_10P_1P8; BUFFER WITH WEAK_PULLDOWN_ON AT 10% SUPPLY VARIATION
IQ_SSDHH_PU_ON_10P_1P8  Cell operated at 1.8(nom)
|IQ_SSDHH_PU_ON_10P_1P8; BUFFER WITH WEAK_PULLUP_ON AT 10% SUPPLY VARIATION
IQ_SSDHH_PUPDOFF_10P_1P8  Cell operated at 1.8(nom)
|IQ_SSDHH_PUPDOFF_10P_1P8; BUFFER WITH WEAK PUPD OFF AT 10% SUPPLY VARIATION
|10% SUPPLY VARIATION MODES WITH 3.3V NOM SUPPLY
IQ_SSDHH_PD_ON_10P_3P3  Cell operated at 3.3(nom)
|IQ_SSDHH_PD_ON_10P_3P3; BUFFER WITH WEAK_PULLDOWN_ON  AT 10% SUPPLY VARIATION
IQ_SSDHH_PU_ON_10P_3P3  Cell operated at 3.3(nom)
|IQ_SSDHH_PU_ON_10P_3P3; BUFFER WITH WEAK_PULLUP_ON AT 10% SUPPLY VARIATION
IQ_SSDHH_PUPDOFF_10P_3P3  Cell operated at 3.3(nom)
|IQ_SSDHH_PUPDOFF_10P_3P3; BUFFER WITH WEAK PUPD OFF AT 10% SUPPLY VARIATION
|   BC1833DV40DCPBFBP18LL_RXLL_SSDLH
[Model Selector] bc1833dv40dcpbfbp18ll_rxll_ssdlh
|SC1 IS A SLEW RATE CONTROL PIN
|5% SUPPLY VARIATION MODES WITH 1.8V NOM SUPPLY
BC40D_H_PUPDOFF_5P_SC1_1P8  Cell operated at 1.8(nom)
|BC40D_H_PUPDOFF_5P_SC1_1P8; BUFFER WITH WEAK PULUP/PULLDOWN OFF AT 5% SUPPLY
|VARIATION WITH SC1=1 MEANING SLOW MODE OF OPERATION
BC40D_H_PD_ON_5P_!SC1_1P8  Cell operated at 1.8(nom)
|BC40D_H_PD_ON_5P_!SC1_1P8; BUFFER WITH WEAK_PULLDOWN_ON AT 5% SUPPLY
|VARIATION WITH SC1=0 MEANING FAST MODE OF OPERATION
BC40D_H_PD_ON_5P_SC1_1P8  Cell operated at 1.8(nom)
|BC40D_H_PD_ON_5P_SC1_1P8; BUFFER WITH WEAK_PULLDOWN_ON AT 5% SUPPLY
|VARIATION WITH SC1=1 MEANING SLOW MODE OF OPERATION
BC40D_H_PU_ON_5P_!SC1_1P8  Cell operated at 1.8(nom)
|BC40D_H_PU_ON_5P_!SC1_1P8; BUFFER WITH WEAK_PULLUP_ON AT 5% SUPPLY
|VARIATION WITH SC1=0 MEANING FAST MODE OF OPERATION
BC40D_H_PUPDOFF_5P_!SC1_1P8  Cell operated at 1.8(nom)
|BC40D_H_PUPDOFF_5P_!SC1_1P8; BUFFER WITH WEAK PULUP/PULLDOWN OFF AT 5% SUPPLY
|VARIATION WITH SC1=0 MEANING FAST MODE OF OPERATION
BC40D_H_PU_ON_5P_SC1_1P8  Cell operated at 1.8(nom)
|BC40D_H_PU_ON_5P_SC1_1P8; BUFFER WITH WEAK_PULLUP_ON AT 5% SUPPLY
|VARIATION WITH SC1=1 MEANING SLOW MODE OF OPERATION
|5% SUPPLY VARIATION MODES WITH 3.3V NOM SUPPLY
BC40D_H_PUPDOFF_5P_SC1_3P3  Cell operated at 3.3(nom)
|BC40D_H_PUPDOFF_5P_SC1_3P3; BUFFER WITH WEAK PULUP/PULLDOWN OFF AT 5% SUPPLY
|VARIATION WITH SC1=1 MEANING SLOW MODE OF OPERATION
BC40D_H_PD_ON_5P_!SC1_3P3  Cell operated at 3.3(nom)
|BC40D_H_PD_ON_5P_!SC1_3P3; BUFFER WITH WEAK_PULLDOWN_ON AT 5% SUPPLY
|VARIATION WITH SC1=0 MEANING FAST MODE OF OPERATION
BC40D_H_PD_ON_5P_SC1_3P3  Cell operated at 3.3(nom)
|BC40D_H_PD_ON_5P_SC1_3P3; BUFFER WITH WEAK_PULLDOWN_ON AT 5% SUPPLY
|VARIATION WITH SC1=1 MEANING SLOW MODE OF OPERATION
BC40D_H_PU_ON_5P_!SC1_3P3  Cell operated at 3.3(nom)
|BC40D_H_PU_ON_5P_!SC1_3P3; BUFFER WITH WEAK_PULLUP_ON AT 5% SUPPLY
|VARIATION WITH SC1=0 MEANING FAST MODE OF OPERATION
BC40D_H_PUPDOFF_5P_!SC1_3P3  Cell operated at 3.3(nom)
|BC40D_H_PUPDOFF_5P_!SC1_3P3; BUFFER WITH WEAK PULUP/PULLDOWN OFF AT 5% SUPPLY
|VARIATION WITH SC1=0 MEANING FAST MODE OF OPERATION
BC40D_H_PU_ON_5P_SC1_3P3  Cell operated at 3.3(nom)
|BC40D_H_PU_ON_5P_SC1_3P3; BUFFER WITH WEAK_PULLUP_ON AT 5% SUPPLY
|VARIATION WITH SC1=1 MEANING SLOW MODE OF OPERATION
| 10% SUPPLY VARIATION MODES WITH 1.8V NOM SUPPLY
BC40D_H_PUPDOFF_10P_SC1_1P8  Cell operated at 1.8(nom)
|BC40D_H_PUPDOFF_10P_SC1_1P8; BUFFER WITH WEAK PULUP/PULLDOWN OFF AT 10% SUPPLY
|VARIATION WITH SC1=1 MEANING SLOW MODE OF OPERATION
BC40D_H_PD_ON_10P_!SC1_1P8  Cell operated at 1.8(nom)
|BC40D_H_PD_ON_10P_!SC1_1P8; BUFFER WITH WEAK_PULLDOWN_ON AT 10% SUPPLY
|VARIATION WITH SC1=0 MEANING FAST MODE OF OPERATION
BC40D_H_PD_ON_10P_SC1_1P8  Cell operated at 1.8(nom)
|BC40D_H_PD_ON_10P_SC1_1P8; BUFFER WITH WEAK_PULLDOWN_ON AT 10% SUPPLY
|VARIATION WITH SC1=1 MEANING SLOW MODE OF OPERATION
BC40D_H_PU_ON_10P_!SC1_1P8  Cell operated at 1.8(nom)
|BC40D_H_PU_ON_10P_!SC1_1P8; BUFFER WITH WEAK_PULLUP_ON AT 10% SUPPLY
|VARIATION WITH SC1=0 MEANING FAST MODE OF OPERATION
BC40D_H_PUPDOFF_10P_!SC1_1P8  Cell operated at 1.8(nom)
|BC40D_H_PUPDOFF_10P_!SC1_1P8; BUFFER WITH WEAK PULUP/PULLDOWN OFF AT 10% SUPPLY
|VARIATION WITH SC1=0 MEANING FAST MODE OF OPERATION
BC40D_H_PU_ON_10P_SC1_1P8  Cell operated at 1.8(nom)
|BC40D_H_PU_ON_10P_SC1_1P8; BUFFER WITH WEAK_PULLUP_ON AT 10% SUPPLY
|VARIATION WITH SC1=1 MEANING SLOW MODE OF OPERATION
| 10% SUPPLY VARIATION MODES WITH 3.3V NOM SUPPLY
BC40D_H_PUPDOFF_10P_SC1_3P3  Cell operated at 3.3(nom)
|BC40D_H_PUPDOFF_10P_SC1_3P3; BUFFER WITH WEAK PULUP/PULLDOWN OFF AT 10% SUPPLY
|VARIATION WITH SC1=1 MEANING SLOW MODE OF OPERATION
BC40D_H_PD_ON_10P_!SC1_3P3  Cell operated at 3.3(nom)
|BC40D_H_PD_ON_10P_!SC1_3P3; BUFFER WITH WEAK_PULLDOWN_ON 10% SUPPLY
|VARIATION WITH SC1=0 MEANING FAST MODE OF OPERATION
BC40D_H_PD_ON_10P_SC1_3P3  Cell operated at 3.3(nom)
|BC40D_H_PD_ON_10P_SC1_3P3; BUFFER WITH WEAK_PULLDOWN_ON AT 10% SUPPLY
|VARIATION WITH SC1=1 MEANING SLOW MODE OF OPERATION
BC40D_H_PU_ON_10P_!SC1_3P3  Cell operated at 3.3(nom)
|BC40D_H_PU_ON_10P_!SC1_3P3; BUFFER WITH WEAK_PULLUP_ON AT 10% SUPPLY
|VARIATION WITH SC1=0 MEANING FAST MODE OF OPERATION
BC40D_H_PUPDOFF_10P_!SC1_3P3  Cell operated at 3.3(nom)
|BC40D_H_PUPDOFF_10P_!SC1_3P3; BUFFER WITH WEAK PULUP/PULLDOWN OFF AT 10% SUPPLY
|VARIATION WITH SC1=0 MEANING FAST MODE OF OPERATION
BC40D_H_PU_ON_10P_SC1_3P3  Cell operated at 3.3(nom)
|BC40D_H_PU_ON_10P_SC1_3P3; BUFFER WITH WEAK_PULLUP_ON AT 10% SUPPLY
|VARIATION WITH SC1=1 MEANING SLOW MODE OF OPERATION
|   BC1833DV40DCPBFBP18LL_RXLL_SSDLV
[Model Selector] bc1833dv40dcpbfbp18ll_rxll_ssdlv
|SC1 IS A SLEW RATE CONTROL PIN
|5% SUPPLY VARIATION MODES WITH 1.8V NOM SUPPLY
BC40D_V_PUPDOFF_5P_SC1_1P8  Cell operated at 1.8(nom)
|BC40D_V_PUPDOFF_5P_SC1_1P8; BUFFER WITH WEAK PULUP/PULLDOWN OFF AT 5% SUPPLY
|VARIATION WITH SC1=1 MEANING SLOW MODE OF OPERATION
BC40D_V_PD_ON_5P_!SC1_1P8  Cell operated at 1.8(nom)
|BC40D_V_PD_ON_5P_!SC1_1P8; BUFFER WITH WEAK_PULLDOWN_ON AT 5% SUPPLY
|VARIATION WITH SC1=0 MEANING FAST MODE OF OPERATION
BC40D_V_PD_ON_5P_SC1_1P8  Cell operated at 1.8(nom)
|BC40D_V_PD_ON_5P_SC1_1P8; BUFFER WITH WEAK_PULLDOWN_ON AT 5% SUPPLY
|VARIATION WITH SC1=1 MEANING SLOW MODE OF OPERATION
BC40D_V_PU_ON_5P_!SC1_1P8  Cell operated at 1.8(nom)
|BC40D_V_PU_ON_5P_!SC1_1P8; BUFFER WITH WEAK_PULLUP_ON AT 5% SUPPLY
|VARIATION WITH SC1=0 MEANING FAST MODE OF OPERATION
BC40D_V_PUPDOFF_5P_!SC1_1P8  Cell operated at 1.8(nom)
|BC40D_V_PUPDOFF_5P_!SC1_1P8; BUFFER WITH WEAK PULUP/PULLDOWN OFF AT 5% SUPPLY
|VARIATION WITH SC1=0 MEANING FAST MODE OF OPERATION
BC40D_V_PU_ON_5P_SC1_1P8  Cell operated at 1.8(nom)
|BC40D_V_PU_ON_5P_SC1_1P8; BUFFER WITH WEAK_PULLUP_ON AT 5% SUPPLY
|VARIATION WITH SC1=1 MEANING SLOW MODE OF OPERATION
|5% SUPPLY VARIATION MODES WITH 3.3V NOM SUPPLY
BC40D_V_PUPDOFF_5P_SC1_3P3  Cell operated at 3.3(nom)
|BC40D_V_PUPDOFF_5P_SC1_3P3; BUFFER WITH WEAK PULUP/PULLDOWN OFF AT 5% SUPPLY
|VARIATION WITH SC1=1 MEANING SLOW MODE OF OPERATION
BC40D_V_PD_ON_5P_!SC1_3P3  Cell operated at 3.3(nom)
|BC40D_V_PD_ON_5P_!SC1_3P3; BUFFER WITH WEAK_PULLDOWN_ON AT 5% SUPPLY
|VARIATION WITH SC1=0 MEANING FAST MODE OF OPERATION
BC40D_V_PD_ON_5P_SC1_3P3  Cell operated at 3.3(nom)
|BC40D_V_PD_ON_5P_SC1_3P3; BUFFER WITH WEAK_PULLDOWN_ON AT 5% SUPPLY
|VARIATION WITH SC1=1 MEANING SLOW MODE OF OPERATION
BC40D_V_PU_ON_5P_!SC1_3P3  Cell operated at 3.3(nom)
|BC40D_V_PU_ON_5P_!SC1_3P3; BUFFER WITH WEAK_PULLUP_ON AT 5% SUPPLY
|VARIATION WITH SC1=0 MEANING FAST MODE OF OPERATION
BC40D_V_PUPDOFF_5P_!SC1_3P3  Cell operated at 3.3(nom)
|BC40D_V_PUPDOFF_5P_!SC1_3P3; BUFFER WITH WEAK PULUP/PULLDOWN OFF AT 5% SUPPLY
|VARIATION WITH SC1=0 MEANING FAST MODE OF OPERATION
BC40D_V_PU_ON_5P_SC1_3P3  Cell operated at 3.3(nom)
|BC40D_V_PU_ON_5P_SC1_3P3; BUFFER WITH WEAK_PULLUP_ON AT 5% SUPPLY
|VARIATION WITH SC1=1 MEANING SLOW MODE OF OPERATION
| 10% SUPPLY VARIATION MODES WITH 1.8V NOM SUPPLY
BC40D_V_PUPDOFF_10P_SC1_1P8  Cell operated at 1.8(nom)
|BC40D_V_PUPDOFF_10P_SC1_1P8; BUFFER WITH WEAK PULUP/PULLDOWN OFF AT 10% SUPPLY
|VARIATION WITH SC1=1 MEANING SLOW MODE OF OPERATION
BC40D_V_PD_ON_10P_!SC1_1P8  Cell operated at 1.8(nom)
|BC40D_V_PD_ON_10P_!SC1_1P8; BUFFER WITH WEAK_PULLDOWN_ON AT 10% SUPPLY
|VARIATION WITH SC1=0 MEANING FAST MODE OF OPERATION
BC40D_V_PD_ON_10P_SC1_1P8  Cell operated at 1.8(nom)
|BC40D_V_PD_ON_10P_SC1_1P8; BUFFER WITH WEAK_PULLDOWN_ON AT 10% SUPPLY
|VARIATION WITH SC1=1 MEANING SLOW MODE OF OPERATION
BC40D_V_PU_ON_10P_!SC1_1P8  Cell operated at 1.8(nom)
|BC40D_V_PU_ON_10P_!SC1_1P8; BUFFER WITH WEAK_PULLUP_ON AT 10% SUPPLY
|VARIATION WITH SC1=0 MEANING FAST MODE OF OPERATION
BC40D_V_PUPDOFF_10P_!SC1_1P8  Cell operated at 1.8(nom)
|BC40D_V_PUPDOFF_10P_!SC1_1P8; BUFFER WITH WEAK PULUP/PULLDOWN OFF AT 10% SUPPLY
|VARIATION WITH SC1=0 MEANING FAST MODE OF OPERATION
BC40D_V_PU_ON_10P_SC1_1P8  Cell operated at 1.8(nom)
|BC40D_V_PU_ON_10P_SC1_1P8; BUFFER WITH WEAK_PULLUP_ON AT 10% SUPPLY
|VARIATION WITH SC1=1 MEANING SLOW MODE OF OPERATION
| 10% SUPPLY VARIATION MODES WITH 3.3V NOM SUPPLY
BC40D_V_PUPDOFF_10P_SC1_3P3  Cell operated at 3.3(nom)
|BC40D_V_PUPDOFF_10P_SC1_3P3; BUFFER WITH WEAK PULUP/PULLDOWN OFF AT 10% SUPPLY
|VARIATION WITH SC1=1 MEANING SLOW MODE OF OPERATION
BC40D_V_PD_ON_10P_!SC1_3P3  Cell operated at 3.3(nom)
|BC40D_V_PD_ON_10P_!SC1_3P3; BUFFER WITH WEAK_PULLDOWN_ON 10% SUPPLY
|VARIATION WITH SC1=0 MEANING FAST MODE OF OPERATION
BC40D_V_PD_ON_10P_SC1_3P3  Cell operated at 3.3(nom)
|BC40D_V_PD_ON_10P_SC1_3P3; BUFFER WITH WEAK_PULLDOWN_ON AT 10% SUPPLY
|VARIATION WITH SC1=1 MEANING SLOW MODE OF OPERATION
BC40D_V_PU_ON_10P_!SC1_3P3  Cell operated at 3.3(nom)
|BC40D_V_PU_ON_10P_!SC1_3P3; BUFFER WITH WEAK_PULLUP_ON AT 10% SUPPLY
|VARIATION WITH SC1=0 MEANING FAST MODE OF OPERATION
BC40D_V_PUPDOFF_10P_!SC1_3P3  Cell operated at 3.3(nom)
|BC40D_V_PUPDOFF_10P_!SC1_3P3; BUFFER WITH WEAK PULUP/PULLDOWN OFF AT 10% SUPPLY
|VARIATION WITH SC1=0 MEANING FAST MODE OF OPERATION
BC40D_V_PU_ON_10P_SC1_3P3  Cell operated at 3.3(nom)
|BC40D_V_PU_ON_10P_SC1_3P3; BUFFER WITH WEAK_PULLUP_ON AT 10% SUPPLY
|VARIATION WITH SC1=1 MEANING SLOW MODE OF OPERATION
|   BC1833DV40DCPBFBP18LL_RXLL_SSDLH_135U
[Model Selector] bc1833dv40dcpbfbp18ll_rxll_ssdlh_135u
|SC1 IS A SLEW RATE CONTROL PIN
|5% SUPPLY VARIATION MODES WITH 1.8V NOM SUPPLY
BC40D_H_PUPDOFF_5P_SC1_1P8  Cell operated at 1.8(nom)
|BC40D_H_PUPDOFF_5P_SC1_1P8; BUFFER WITH WEAK PULUP/PULLDOWN OFF AT 5% SUPPLY
|VARIATION WITH SC1=1 MEANING SLOW MODE OF OPERATION
BC40D_H_PD_ON_5P_!SC1_1P8  Cell operated at 1.8(nom)
|BC40D_H_PD_ON_5P_!SC1_1P8; BUFFER WITH WEAK_PULLDOWN_ON AT 5% SUPPLY
|VARIATION WITH SC1=0 MEANING FAST MODE OF OPERATION
BC40D_H_PD_ON_5P_SC1_1P8  Cell operated at 1.8(nom)
|BC40D_H_PD_ON_5P_SC1_1P8; BUFFER WITH WEAK_PULLDOWN_ON AT 5% SUPPLY
|VARIATION WITH SC1=1 MEANING SLOW MODE OF OPERATION
BC40D_H_PU_ON_5P_!SC1_1P8  Cell operated at 1.8(nom)
|BC40D_H_PU_ON_5P_!SC1_1P8; BUFFER WITH WEAK_PULLUP_ON AT 5% SUPPLY
|VARIATION WITH SC1=0 MEANING FAST MODE OF OPERATION
BC40D_H_PUPDOFF_5P_!SC1_1P8  Cell operated at 1.8(nom)
|BC40D_H_PUPDOFF_5P_!SC1_1P8; BUFFER WITH WEAK PULUP/PULLDOWN OFF AT 5% SUPPLY
|VARIATION WITH SC1=0 MEANING FAST MODE OF OPERATION
BC40D_H_PU_ON_5P_SC1_1P8  Cell operated at 1.8(nom)
|BC40D_H_PU_ON_5P_SC1_1P8; BUFFER WITH WEAK_PULLUP_ON AT 5% SUPPLY
|VARIATION WITH SC1=1 MEANING SLOW MODE OF OPERATION
|5% SUPPLY VARIATION MODES WITH 3.3V NOM SUPPLY
BC40D_H_PUPDOFF_5P_SC1_3P3  Cell operated at 3.3(nom)
|BC40D_H_PUPDOFF_5P_SC1_3P3; BUFFER WITH WEAK PULUP/PULLDOWN OFF AT 5% SUPPLY
|VARIATION WITH SC1=1 MEANING SLOW MODE OF OPERATION
BC40D_H_PD_ON_5P_!SC1_3P3  Cell operated at 3.3(nom)
|BC40D_H_PD_ON_5P_!SC1_3P3; BUFFER WITH WEAK_PULLDOWN_ON AT 5% SUPPLY
|VARIATION WITH SC1=0 MEANING FAST MODE OF OPERATION
BC40D_H_PD_ON_5P_SC1_3P3  Cell operated at 3.3(nom)
|BC40D_H_PD_ON_5P_SC1_3P3; BUFFER WITH WEAK_PULLDOWN_ON AT 5% SUPPLY
|VARIATION WITH SC1=1 MEANING SLOW MODE OF OPERATION
BC40D_H_PU_ON_5P_!SC1_3P3  Cell operated at 3.3(nom)
|BC40D_H_PU_ON_5P_!SC1_3P3; BUFFER WITH WEAK_PULLUP_ON AT 5% SUPPLY
|VARIATION WITH SC1=0 MEANING FAST MODE OF OPERATION
BC40D_H_PUPDOFF_5P_!SC1_3P3  Cell operated at 3.3(nom)
|BC40D_H_PUPDOFF_5P_!SC1_3P3; BUFFER WITH WEAK PULUP/PULLDOWN OFF AT 5% SUPPLY
|VARIATION WITH SC1=0 MEANING FAST MODE OF OPERATION
BC40D_H_PU_ON_5P_SC1_3P3  Cell operated at 3.3(nom)
|BC40D_H_PU_ON_5P_SC1_3P3; BUFFER WITH WEAK_PULLUP_ON AT 5% SUPPLY
|VARIATION WITH SC1=1 MEANING SLOW MODE OF OPERATION
| 10% SUPPLY VARIATION MODES WITH 1.8V NOM SUPPLY
BC40D_H_PUPDOFF_10P_SC1_1P8  Cell operated at 1.8(nom)
|BC40D_H_PUPDOFF_10P_SC1_1P8; BUFFER WITH WEAK PULUP/PULLDOWN OFF AT 10% SUPPLY
|VARIATION WITH SC1=1 MEANING SLOW MODE OF OPERATION
BC40D_H_PD_ON_10P_!SC1_1P8  Cell operated at 1.8(nom)
|BC40D_H_PD_ON_10P_!SC1_1P8; BUFFER WITH WEAK_PULLDOWN_ON AT 10% SUPPLY
|VARIATION WITH SC1=0 MEANING FAST MODE OF OPERATION
BC40D_H_PD_ON_10P_SC1_1P8  Cell operated at 1.8(nom)
|BC40D_H_PD_ON_10P_SC1_1P8; BUFFER WITH WEAK_PULLDOWN_ON AT 10% SUPPLY
|VARIATION WITH SC1=1 MEANING SLOW MODE OF OPERATION
BC40D_H_PU_ON_10P_!SC1_1P8  Cell operated at 1.8(nom)
|BC40D_H_PU_ON_10P_!SC1_1P8; BUFFER WITH WEAK_PULLUP_ON AT 10% SUPPLY
|VARIATION WITH SC1=0 MEANING FAST MODE OF OPERATION
BC40D_H_PUPDOFF_10P_!SC1_1P8  Cell operated at 1.8(nom)
|BC40D_H_PUPDOFF_10P_!SC1_1P8; BUFFER WITH WEAK PULUP/PULLDOWN OFF AT 10% SUPPLY
|VARIATION WITH SC1=0 MEANING FAST MODE OF OPERATION
BC40D_H_PU_ON_10P_SC1_1P8  Cell operated at 1.8(nom)
|BC40D_H_PU_ON_10P_SC1_1P8; BUFFER WITH WEAK_PULLUP_ON AT 10% SUPPLY
|VARIATION WITH SC1=1 MEANING SLOW MODE OF OPERATION
| 10% SUPPLY VARIATION MODES WITH 3.3V NOM SUPPLY
BC40D_H_PUPDOFF_10P_SC1_3P3  Cell operated at 3.3(nom)
|BC40D_H_PUPDOFF_10P_SC1_3P3; BUFFER WITH WEAK PULUP/PULLDOWN OFF AT 10% SUPPLY
|VARIATION WITH SC1=1 MEANING SLOW MODE OF OPERATION
BC40D_H_PD_ON_10P_!SC1_3P3  Cell operated at 3.3(nom)
|BC40D_H_PD_ON_10P_!SC1_3P3; BUFFER WITH WEAK_PULLDOWN_ON 10% SUPPLY
|VARIATION WITH SC1=0 MEANING FAST MODE OF OPERATION
BC40D_H_PD_ON_10P_SC1_3P3  Cell operated at 3.3(nom)
|BC40D_H_PD_ON_10P_SC1_3P3; BUFFER WITH WEAK_PULLDOWN_ON AT 10% SUPPLY
|VARIATION WITH SC1=1 MEANING SLOW MODE OF OPERATION
BC40D_H_PU_ON_10P_!SC1_3P3  Cell operated at 3.3(nom)
|BC40D_H_PU_ON_10P_!SC1_3P3; BUFFER WITH WEAK_PULLUP_ON AT 10% SUPPLY
|VARIATION WITH SC1=0 MEANING FAST MODE OF OPERATION
BC40D_H_PUPDOFF_10P_!SC1_3P3  Cell operated at 3.3(nom)
|BC40D_H_PUPDOFF_10P_!SC1_3P3; BUFFER WITH WEAK PULUP/PULLDOWN OFF AT 10% SUPPLY
|VARIATION WITH SC1=0 MEANING FAST MODE OF OPERATION
BC40D_H_PU_ON_10P_SC1_3P3  Cell operated at 3.3(nom)
|BC40D_H_PU_ON_10P_SC1_3P3; BUFFER WITH WEAK_PULLUP_ON AT 10% SUPPLY
|VARIATION WITH SC1=1 MEANING SLOW MODE OF OPERATION
|   BC1833DV40DCPBFBP18LL_RXLL_SSDLV_135U
[Model Selector] bc1833dv40dcpbfbp18ll_rxll_ssdlv_135u
|SC1 IS A SLEW RATE CONTROL PIN
|5% SUPPLY VARIATION MODES WITH 1.8V NOM SUPPLY
BC40D_V_PUPDOFF_5P_SC1_1P8  Cell operated at 1.8(nom)
|BC40D_V_PUPDOFF_5P_SC1_1P8; BUFFER WITH WEAK PULUP/PULLDOWN OFF AT 5% SUPPLY
|VARIATION WITH SC1=1 MEANING SLOW MODE OF OPERATION
BC40D_V_PD_ON_5P_!SC1_1P8  Cell operated at 1.8(nom)
|BC40D_V_PD_ON_5P_!SC1_1P8; BUFFER WITH WEAK_PULLDOWN_ON AT 5% SUPPLY
|VARIATION WITH SC1=0 MEANING FAST MODE OF OPERATION
BC40D_V_PD_ON_5P_SC1_1P8  Cell operated at 1.8(nom)
|BC40D_V_PD_ON_5P_SC1_1P8; BUFFER WITH WEAK_PULLDOWN_ON AT 5% SUPPLY
|VARIATION WITH SC1=1 MEANING SLOW MODE OF OPERATION
BC40D_V_PU_ON_5P_!SC1_1P8  Cell operated at 1.8(nom)
|BC40D_V_PU_ON_5P_!SC1_1P8; BUFFER WITH WEAK_PULLUP_ON AT 5% SUPPLY
|VARIATION WITH SC1=0 MEANING FAST MODE OF OPERATION
BC40D_V_PUPDOFF_5P_!SC1_1P8  Cell operated at 1.8(nom)
|BC40D_V_PUPDOFF_5P_!SC1_1P8; BUFFER WITH WEAK PULUP/PULLDOWN OFF AT 5% SUPPLY
|VARIATION WITH SC1=0 MEANING FAST MODE OF OPERATION
BC40D_V_PU_ON_5P_SC1_1P8  Cell operated at 1.8(nom)
|BC40D_V_PU_ON_5P_SC1_1P8; BUFFER WITH WEAK_PULLUP_ON AT 5% SUPPLY
|VARIATION WITH SC1=1 MEANING SLOW MODE OF OPERATION
|5% SUPPLY VARIATION MODES WITH 3.3V NOM SUPPLY
BC40D_V_PUPDOFF_5P_SC1_3P3  Cell operated at 3.3(nom)
|BC40D_V_PUPDOFF_5P_SC1_3P3; BUFFER WITH WEAK PULUP/PULLDOWN OFF AT 5% SUPPLY
|VARIATION WITH SC1=1 MEANING SLOW MODE OF OPERATION
BC40D_V_PD_ON_5P_!SC1_3P3  Cell operated at 3.3(nom)
|BC40D_V_PD_ON_5P_!SC1_3P3; BUFFER WITH WEAK_PULLDOWN_ON AT 5% SUPPLY
|VARIATION WITH SC1=0 MEANING FAST MODE OF OPERATION
BC40D_V_PD_ON_5P_SC1_3P3  Cell operated at 3.3(nom)
|BC40D_V_PD_ON_5P_SC1_3P3; BUFFER WITH WEAK_PULLDOWN_ON AT 5% SUPPLY
|VARIATION WITH SC1=1 MEANING SLOW MODE OF OPERATION
BC40D_V_PU_ON_5P_!SC1_3P3  Cell operated at 3.3(nom)
|BC40D_V_PU_ON_5P_!SC1_3P3; BUFFER WITH WEAK_PULLUP_ON AT 5% SUPPLY
|VARIATION WITH SC1=0 MEANING FAST MODE OF OPERATION
BC40D_V_PUPDOFF_5P_!SC1_3P3  Cell operated at 3.3(nom)
|BC40D_V_PUPDOFF_5P_!SC1_3P3; BUFFER WITH WEAK PULUP/PULLDOWN OFF AT 5% SUPPLY
|VARIATION WITH SC1=0 MEANING FAST MODE OF OPERATION
BC40D_V_PU_ON_5P_SC1_3P3  Cell operated at 3.3(nom)
|BC40D_V_PU_ON_5P_SC1_3P3; BUFFER WITH WEAK_PULLUP_ON AT 5% SUPPLY
|VARIATION WITH SC1=1 MEANING SLOW MODE OF OPERATION
| 10% SUPPLY VARIATION MODES WITH 1.8V NOM SUPPLY
BC40D_V_PUPDOFF_10P_SC1_1P8  Cell operated at 1.8(nom)
|BC40D_V_PUPDOFF_10P_SC1_1P8; BUFFER WITH WEAK PULUP/PULLDOWN OFF AT 10% SUPPLY
|VARIATION WITH SC1=1 MEANING SLOW MODE OF OPERATION
BC40D_V_PD_ON_10P_!SC1_1P8  Cell operated at 1.8(nom)
|BC40D_V_PD_ON_10P_!SC1_1P8; BUFFER WITH WEAK_PULLDOWN_ON AT 10% SUPPLY
|VARIATION WITH SC1=0 MEANING FAST MODE OF OPERATION
BC40D_V_PD_ON_10P_SC1_1P8  Cell operated at 1.8(nom)
|BC40D_V_PD_ON_10P_SC1_1P8; BUFFER WITH WEAK_PULLDOWN_ON AT 10% SUPPLY
|VARIATION WITH SC1=1 MEANING SLOW MODE OF OPERATION
BC40D_V_PU_ON_10P_!SC1_1P8  Cell operated at 1.8(nom)
|BC40D_V_PU_ON_10P_!SC1_1P8; BUFFER WITH WEAK_PULLUP_ON AT 10% SUPPLY
|VARIATION WITH SC1=0 MEANING FAST MODE OF OPERATION
BC40D_V_PUPDOFF_10P_!SC1_1P8  Cell operated at 1.8(nom)
|BC40D_V_PUPDOFF_10P_!SC1_1P8; BUFFER WITH WEAK PULUP/PULLDOWN OFF AT 10% SUPPLY
|VARIATION WITH SC1=0 MEANING FAST MODE OF OPERATION
BC40D_V_PU_ON_10P_SC1_1P8  Cell operated at 1.8(nom)
|BC40D_V_PU_ON_10P_SC1_1P8; BUFFER WITH WEAK_PULLUP_ON AT 10% SUPPLY
|VARIATION WITH SC1=1 MEANING SLOW MODE OF OPERATION
| 10% SUPPLY VARIATION MODES WITH 3.3V NOM SUPPLY
BC40D_V_PUPDOFF_10P_SC1_3P3  Cell operated at 3.3(nom)
|BC40D_V_PUPDOFF_10P_SC1_3P3; BUFFER WITH WEAK PULUP/PULLDOWN OFF AT 10% SUPPLY
|VARIATION WITH SC1=1 MEANING SLOW MODE OF OPERATION
BC40D_V_PD_ON_10P_!SC1_3P3  Cell operated at 3.3(nom)
|BC40D_V_PD_ON_10P_!SC1_3P3; BUFFER WITH WEAK_PULLDOWN_ON 10% SUPPLY
|VARIATION WITH SC1=0 MEANING FAST MODE OF OPERATION
BC40D_V_PD_ON_10P_SC1_3P3  Cell operated at 3.3(nom)
|BC40D_V_PD_ON_10P_SC1_3P3; BUFFER WITH WEAK_PULLDOWN_ON AT 10% SUPPLY
|VARIATION WITH SC1=1 MEANING SLOW MODE OF OPERATION
BC40D_V_PU_ON_10P_!SC1_3P3  Cell operated at 3.3(nom)
|BC40D_V_PU_ON_10P_!SC1_3P3; BUFFER WITH WEAK_PULLUP_ON AT 10% SUPPLY
|VARIATION WITH SC1=0 MEANING FAST MODE OF OPERATION
BC40D_V_PUPDOFF_10P_!SC1_3P3  Cell operated at 3.3(nom)
|BC40D_V_PUPDOFF_10P_!SC1_3P3; BUFFER WITH WEAK PULUP/PULLDOWN OFF AT 10% SUPPLY
|VARIATION WITH SC1=0 MEANING FAST MODE OF OPERATION
BC40D_V_PU_ON_10P_SC1_3P3  Cell operated at 3.3(nom)
|BC40D_V_PU_ON_10P_SC1_3P3; BUFFER WITH WEAK_PULLUP_ON AT 10% SUPPLY
|VARIATION WITH SC1=1 MEANING SLOW MODE OF OPERATION
|   BC1833DV40DCPBFBP18LL_SSDLH_135U
[Model Selector] bc1833dv40dcpbfbp18ll_ssdlh_135u
|SC1 IS A SLEW RATE CONTROL PIN
|5% SUPPLY VARIATION MODES WITH 1.8V NOM SUPPLY
BC40D_H_PUPDOFF_5P_SC1_1P8  Cell operated at 1.8(nom)
|BC40D_H_PUPDOFF_5P_SC1_1P8; BUFFER WITH WEAK PULUP/PULLDOWN OFF AT 5% SUPPLY
|VARIATION WITH SC1=1 MEANING SLOW MODE OF OPERATION
BC40D_H_PD_ON_5P_!SC1_1P8  Cell operated at 1.8(nom)
|BC40D_H_PD_ON_5P_!SC1_1P8; BUFFER WITH WEAK_PULLDOWN_ON AT 5% SUPPLY
|VARIATION WITH SC1=0 MEANING FAST MODE OF OPERATION
BC40D_H_PD_ON_5P_SC1_1P8  Cell operated at 1.8(nom)
|BC40D_H_PD_ON_5P_SC1_1P8; BUFFER WITH WEAK_PULLDOWN_ON AT 5% SUPPLY
|VARIATION WITH SC1=1 MEANING SLOW MODE OF OPERATION
BC40D_H_PU_ON_5P_!SC1_1P8  Cell operated at 1.8(nom)
|BC40D_H_PU_ON_5P_!SC1_1P8; BUFFER WITH WEAK_PULLUP_ON AT 5% SUPPLY
|VARIATION WITH SC1=0 MEANING FAST MODE OF OPERATION
BC40D_H_PUPDOFF_5P_!SC1_1P8  Cell operated at 1.8(nom)
|BC40D_H_PUPDOFF_5P_!SC1_1P8; BUFFER WITH WEAK PULUP/PULLDOWN OFF AT 5% SUPPLY
|VARIATION WITH SC1=0 MEANING FAST MODE OF OPERATION
BC40D_H_PU_ON_5P_SC1_1P8  Cell operated at 1.8(nom)
|BC40D_H_PU_ON_5P_SC1_1P8; BUFFER WITH WEAK_PULLUP_ON AT 5% SUPPLY
|VARIATION WITH SC1=1 MEANING SLOW MODE OF OPERATION
|5% SUPPLY VARIATION MODES WITH 3.3V NOM SUPPLY
BC40D_H_PUPDOFF_5P_SC1_3P3  Cell operated at 3.3(nom)
|BC40D_H_PUPDOFF_5P_SC1_3P3; BUFFER WITH WEAK PULUP/PULLDOWN OFF AT 5% SUPPLY
|VARIATION WITH SC1=1 MEANING SLOW MODE OF OPERATION
BC40D_H_PD_ON_5P_!SC1_3P3  Cell operated at 3.3(nom)
|BC40D_H_PD_ON_5P_!SC1_3P3; BUFFER WITH WEAK_PULLDOWN_ON AT 5% SUPPLY
|VARIATION WITH SC1=0 MEANING FAST MODE OF OPERATION
BC40D_H_PD_ON_5P_SC1_3P3  Cell operated at 3.3(nom)
|BC40D_H_PD_ON_5P_SC1_3P3; BUFFER WITH WEAK_PULLDOWN_ON AT 5% SUPPLY
|VARIATION WITH SC1=1 MEANING SLOW MODE OF OPERATION
BC40D_H_PU_ON_5P_!SC1_3P3  Cell operated at 3.3(nom)
|BC40D_H_PU_ON_5P_!SC1_3P3; BUFFER WITH WEAK_PULLUP_ON AT 5% SUPPLY
|VARIATION WITH SC1=0 MEANING FAST MODE OF OPERATION
BC40D_H_PUPDOFF_5P_!SC1_3P3  Cell operated at 3.3(nom)
|BC40D_H_PUPDOFF_5P_!SC1_3P3; BUFFER WITH WEAK PULUP/PULLDOWN OFF AT 5% SUPPLY
|VARIATION WITH SC1=0 MEANING FAST MODE OF OPERATION
BC40D_H_PU_ON_5P_SC1_3P3  Cell operated at 3.3(nom)
|BC40D_H_PU_ON_5P_SC1_3P3; BUFFER WITH WEAK_PULLUP_ON AT 5% SUPPLY
|VARIATION WITH SC1=1 MEANING SLOW MODE OF OPERATION
| 10% SUPPLY VARIATION MODES WITH 1.8V NOM SUPPLY
BC40D_H_PUPDOFF_10P_SC1_1P8  Cell operated at 1.8(nom)
|BC40D_H_PUPDOFF_10P_SC1_1P8; BUFFER WITH WEAK PULUP/PULLDOWN OFF AT 10% SUPPLY
|VARIATION WITH SC1=1 MEANING SLOW MODE OF OPERATION
BC40D_H_PD_ON_10P_!SC1_1P8  Cell operated at 1.8(nom)
|BC40D_H_PD_ON_10P_!SC1_1P8; BUFFER WITH WEAK_PULLDOWN_ON AT 10% SUPPLY
|VARIATION WITH SC1=0 MEANING FAST MODE OF OPERATION
BC40D_H_PD_ON_10P_SC1_1P8  Cell operated at 1.8(nom)
|BC40D_H_PD_ON_10P_SC1_1P8; BUFFER WITH WEAK_PULLDOWN_ON AT 10% SUPPLY
|VARIATION WITH SC1=1 MEANING SLOW MODE OF OPERATION
BC40D_H_PU_ON_10P_!SC1_1P8  Cell operated at 1.8(nom)
|BC40D_H_PU_ON_10P_!SC1_1P8; BUFFER WITH WEAK_PULLUP_ON AT 10% SUPPLY
|VARIATION WITH SC1=0 MEANING FAST MODE OF OPERATION
BC40D_H_PUPDOFF_10P_!SC1_1P8  Cell operated at 1.8(nom)
|BC40D_H_PUPDOFF_10P_!SC1_1P8; BUFFER WITH WEAK PULUP/PULLDOWN OFF AT 10% SUPPLY
|VARIATION WITH SC1=0 MEANING FAST MODE OF OPERATION
BC40D_H_PU_ON_10P_SC1_1P8  Cell operated at 1.8(nom)
|BC40D_H_PU_ON_10P_SC1_1P8; BUFFER WITH WEAK_PULLUP_ON AT 10% SUPPLY
|VARIATION WITH SC1=1 MEANING SLOW MODE OF OPERATION
| 10% SUPPLY VARIATION MODES WITH 3.3V NOM SUPPLY
BC40D_H_PUPDOFF_10P_SC1_3P3  Cell operated at 3.3(nom)
|BC40D_H_PUPDOFF_10P_SC1_3P3; BUFFER WITH WEAK PULUP/PULLDOWN OFF AT 10% SUPPLY
|VARIATION WITH SC1=1 MEANING SLOW MODE OF OPERATION
BC40D_H_PD_ON_10P_!SC1_3P3  Cell operated at 3.3(nom)
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| Models and submodels in the file (68): BC40D_H_PUPDOFF_5P_SC1_1P8 (I/O), BC40D_H_PD_ON_5P_!SC1_1P8 (I/O), BC40D_H_PD_ON_5P_SC1_1P8 (I/O), BC40D_H_PU_ON_5P_!SC1_1P8 (I/O), BC40D_H_PUPDOFF_5P_!SC1_1P8 (I/O), BC40D_H_PU_ON_5P_SC1_1P8 (I/O), BC40D_H_PUPDOFF_5P_SC1_3P3 (I/O), BC40D_H_PD_ON_5P_!SC1_3P3 (I/O), BC40D_H_PD_ON_5P_SC1_3P3 (I/O), BC40D_H_PU_ON_5P_!SC1_3P3 (I/O), BC40D_H_PUPDOFF_5P_!SC1_3P3 (I/O), BC40D_H_PU_ON_5P_SC1_3P3 (I/O), BC40D_H_PUPDOFF_10P_SC1_1P8 (I/O), BC40D_H_PD_ON_10P_!SC1_1P8 (I/O), BC40D_H_PD_ON_10P_SC1_1P8 (I/O), BC40D_H_PU_ON_10P_!SC1_1P8 (I/O), BC40D_H_PUPDOFF_10P_!SC1_1P8 (I/O), BC40D_H_PU_ON_10P_SC1_1P8 (I/O), BC40D_H_PUPDOFF_10P_SC1_3P3 (I/O), BC40D_H_PD_ON_10P_!SC1_3P3 (I/O), BC40D_H_PD_ON_10P_SC1_3P3 (I/O), BC40D_H_PU_ON_10P_!SC1_3P3 (I/O), BC40D_H_PUPDOFF_10P_!SC1_3P3 (I/O), BC40D_H_PU_ON_10P_SC1_3P3 (I/O), BC40D_V_PUPDOFF_5P_SC1_1P8 (I/O), BC40D_V_PD_ON_5P_!SC1_1P8 (I/O), BC40D_V_PD_ON_5P_SC1_1P8 (I/O), BC40D_V_PU_ON_5P_!SC1_1P8 (I/O), BC40D_V_PUPDOFF_5P_!SC1_1P8 (I/O), BC40D_V_PU_ON_5P_SC1_1P8 (I/O), BC40D_V_PUPDOFF_5P_SC1_3P3 (I/O), BC40D_V_PD_ON_5P_!SC1_3P3 (I/O), BC40D_V_PD_ON_5P_SC1_3P3 (I/O), BC40D_V_PU_ON_5P_!SC1_3P3 (I/O), BC40D_V_PUPDOFF_5P_!SC1_3P3 (I/O), BC40D_V_PU_ON_5P_SC1_3P3 (I/O), BC40D_V_PUPDOFF_10P_SC1_1P8 (I/O), BC40D_V_PD_ON_10P_!SC1_1P8 (I/O), BC40D_V_PD_ON_10P_SC1_1P8 (I/O), BC40D_V_PU_ON_10P_!SC1_1P8 (I/O), BC40D_V_PUPDOFF_10P_!SC1_1P8 (I/O), BC40D_V_PU_ON_10P_SC1_1P8 (I/O), BC40D_V_PUPDOFF_10P_SC1_3P3 (I/O), BC40D_V_PD_ON_10P_!SC1_3P3 (I/O), BC40D_V_PD_ON_10P_SC1_3P3 (I/O), BC40D_V_PU_ON_10P_!SC1_3P3 (I/O), BC40D_V_PUPDOFF_10P_!SC1_3P3 (I/O), BC40D_V_PU_ON_10P_SC1_3P3 (I/O), BI2C1833_NORAML_5P_1P8 (I/O_open_drain), BI2C1833_NORAML_5P_3P3 (I/O_open_drain), BI2C1833_NORAML_10P_1P8 (I/O_open_drain), BI2C1833_NORAML_10P_3P3 (I/O_open_drain), IHHV_NORAML_5P_1P8 (Input), IHHV_NORAML_5P_3P3 (Input), IHHV_NORAML_10P_1P8 (Input), IHHV_NORAML_10P_3P3 (Input), IQ_SSDHH_PD_ON_5P_1P8 (Input), IQ_SSDHH_PU_ON_5P_1P8 (Input), IQ_SSDHH_PUPDOFF_5P_1P8 (Input), IQ_SSDHH_PD_ON_5P_3P3 (Input), IQ_SSDHH_PU_ON_5P_3P3 (Input), IQ_SSDHH_PUPDOFF_5P_3P3 (Input), IQ_SSDHH_PD_ON_10P_1P8 (Input), IQ_SSDHH_PU_ON_10P_1P8 (Input), IQ_SSDHH_PUPDOFF_10P_1P8 (Input), IQ_SSDHH_PD_ON_10P_3P3 (Input), IQ_SSDHH_PU_ON_10P_3P3 (Input), IQ_SSDHH_PUPDOFF_10P_3P3 (Input)
